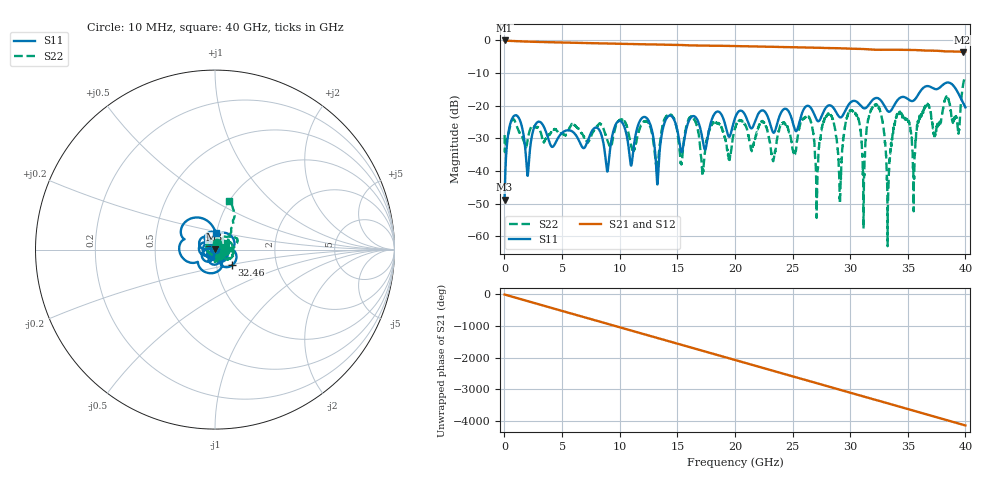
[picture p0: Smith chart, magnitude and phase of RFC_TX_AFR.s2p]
!Keysight Technologies,N5245B,MY57181321,A.13.80.12
!Automatic Fixture Removal (AFR)
!Date: Tuesday, May 12, 2020, 04:32:56
!S2P File: Measurements: S11,S21,S12,S22:
# MHz S  RI  R 50
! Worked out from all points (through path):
!   4000 points, 10 MHz to 40 GHz, reference 50 ohm
!   highest |S21| = -0.03 dB at 10 MHz (marker M1); lowest = -3.5 dB at 39.76 GHz (marker M2)
!   group delay of S21, straight-line fit = 287 ps
!   lowest |S11| = -48.8 dB at 10 MHz (marker M3), VSWR 1.01, Z = 49.7 + j0.258 ohm
!   |S11| at or under -10 dB: start of sweep to end of sweep
!   |S22| runs from -63.0 to -10.9 dB; largest |S21 - S12| = 1.5e-15
!   S11 on the Smith chart (normalised r, x): 10 MHz: 0.99, +0.01; 32.46 GHz: 1.19, -0.21; 40 GHz: 0.99, +0.19
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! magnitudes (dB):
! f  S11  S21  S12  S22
! 10 MHz  -48.8  0.0  0.0  -29.0
! 890 MHz  -23.0  -0.3  -0.3  -24.6
! 2 GHz  -41.5  -0.4  -0.4  -30.8
! 2.93 GHz  -24.9  -0.5  -0.5  -26.6
! 6.68 GHz  -32.3  -0.8  -0.8  -28.3
! 12.19 GHz  -23.5  -1.2  -1.2  -24.8
! 13.34 GHz  -40.5  -1.3  -1.3  -37.0
! 14.25 GHz  -23.1  -1.4  -1.4  -22.7
! 17.21 GHz  -30.8  -1.6  -1.6  -40.4
! 20.01 GHz  -23.7  -1.7  -1.7  -26.9
! 26.67 GHz  -21.1  -2.2  -2.2  -25.9
! 27.12 GHz  -24.5  -2.3  -2.3  -48.0
! 28.31 GHz  -19.9  -2.4  -2.4  -22.8
! 29.13 GHz  -23.6  -2.4  -2.4  -47.4
! 29.91 GHz  -19.5  -2.5  -2.5  -21.8
! 31.17 GHz  -20.8  -2.7  -2.7  -51.9
! 32.46 GHz  -17.8  -2.9  -2.9  -20.7
! 33.34 GHz  -21.8  -2.9  -2.9  -41.8
! 34.16 GHz  -18.1  -2.9  -2.9  -22.2
! 35.52 GHz  -18.4  -3.0  -3.0  -45.5
! 39.76 GHz  -18.8  -3.5  -3.5  -14.4
! 40 GHz  -20.5  -3.4  -3.4  -10.9
